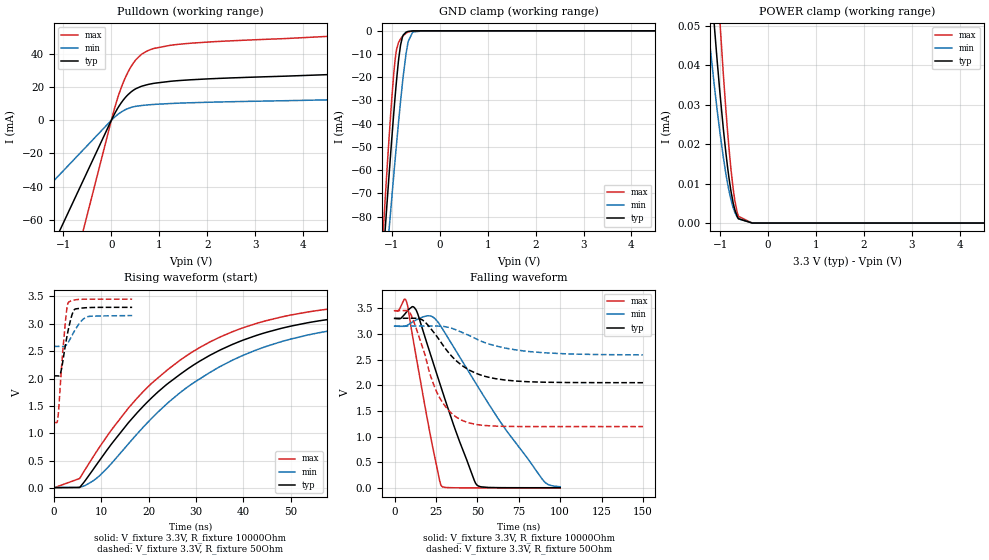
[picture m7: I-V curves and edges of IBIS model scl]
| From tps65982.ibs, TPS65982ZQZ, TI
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|   scl Model
[Model]   scl
Model_type   I/O_open_drain
Polarity   Non-Inverting
Vinl = 0.80
Vinh = 2.00
Vmeas = 1.65
Vref = 3.3
Cref = 2pF
Rref = 10000
|   typ   min   max
|   (nom PVT)   (fast PVT)   (slow PVT)
C_comp   8.631e-13   8.505e-13   8.892e-13
| Where nom  PVT is Nominal Process, 3.3V, 27C
|   Fast PVT is Strong Process,  3.45V, -40C
|   Slow PVT is Weak Process,   3.15V, 125C
[Voltage Range]   3.3   3.15   3.45
|Junction Temperature
[Temperature Range]   27   125   -40
[Pullup Reference]   3.3   3.15   3.45
[Pulldown Reference]   0   0   0
[Power Clamp Reference]   3.3   3.15   3.45
[GND Clamp Reference]   0   0   0
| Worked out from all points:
|   slope of the pulldown table from 0 to 0.495 V, typ, clamps not added: 26.4 ohm
|   GND clamp passes 1 mA (typ) near -0.72 V on its own axis
|   falling waveform, V_fixture 3.3V, R_fixture 10000Ohm: 20-80 % time 20.9ns typ, 38.8ns min, 11.8ns max; typ from 3.3 V to 0.005 V
|   rising waveform, V_fixture 3.3V, R_fixture 10000Ohm: 20-80 % time 26.8ns typ, 28.1ns min, 25.7ns max; typ from 0.005 V to 3.28 V
|   falling waveform, V_fixture 3.3V, R_fixture 50Ohm: 20-80 % time 21.7ns typ, 30.6ns min, 15.2ns max; typ from 3.3 V to 2.05 V
|   rising waveform, V_fixture 3.3V, R_fixture 50Ohm: 20-80 % time 1.6ns typ, 2.37ns min, 1.21ns max; typ from 2.05 V to 3.3 V
[Pulldown]
|   Voltage   I(typ)   I(min)   I(max)
-3.3V     -204.1mA   -100.3mA   -374.1mA
-55.5mV   -3.433mA   -1.687mA   -6.291mA
63.75mV   3.72mA     1.782mA    6.922mA
132.8mV   7.276mA    3.46mA     13.56mA
308.7mV   14.28mA    6.613mA    26.84mA
412.2mV   17.12mA    7.756mA    32.46mA
519.2mV   19.17mA    8.464mA    36.77mA
753.8mV   21.53mA    9.255mA    41.92mA
1.251V    23.57mA    10.13mA    45.33mA
1.645V    24.41mA    10.56mA    46.48mA
5.363V    28.43mA    12.81mA    51.9mA
6.6V      30.97mA    14.1mA     56.05mA
[GND Clamp]
|   Voltage   I(typ)   I(min)   I(max)
-3.3V     -769.8mA   -681.9mA   -862.9mA
-1.224V   -111.3mA   -127.9mA   -102mA
-1.109V   -77.43mA   -98.96mA   -63.21mA
-1.051V   -60.73mA   -84.56mA   -44.53mA
-964.4mV  -37.15mA   -63.69mA   -19.94mA
-912.3mV  -24.19mA   -51.54mA   -9.676mA
-815.1mV  -5.994mA   -30.18mA   -3.458mA
-701.3mV  -575.2uA   -9.847mA   -1.031mA
-653.9mV  -240.8uA   -4.467mA   -490.7uA
-562.6mV  -38.43uA   -514.1uA   -74.23uA
-330mV    -101.2nA   -940.3nA   -65.96nA
6.6V      0A         0A         0A
[POWER Clamp]
|   Voltage   I(typ)   I(min)   I(max)
-3.3V     548.7uA    403.1uA    721.8uA
-1.299V   79.98uA    55.9uA     116.4uA
-1.208V   64.23uA    44.79uA    94.82uA
-1.111V   48.63uA    33.84uA    73.12uA
-1.004V   33.07uA    23.01uA    51.08uA
-881.5mV  18.07uA    12.69uA    29.13uA
-815.1mV  11.51uA    8.232uA    19.09uA
-774.6mV  8.211uA    6.002uA    13.83uA
-695.3mV  3.499uA    2.796uA    5.93uA
-615.9mV  1.099uA    1.051uA    1.702uA
-330mV    0A         10.54nA    0A
6.6V      0A         0A         0A
[Ramp]
R_load = 10000
|   typ   min   max
dV/dt_r   1.96448/2.6802e-08   1.86581/2.80237e-08   2.05933/2.56593e-08
dV/dt_f   1.97678/2.08974e-08   1.87506/3.88653e-08   2.06819/1.17648e-08
[Falling Waveform]
V_fixture = 3.3V
V_fixture_min = 3.15V
V_fixture_max = 3.45V
R_fixture = 10000Ohm
|   Time   V(typ)   V(min)   V(max)
0s        3.3V       3.15V      3.45V
2.424ns   3.294V     3.145V     3.453V
5.864ns   3.371V     3.145V     3.673V
7.472ns   3.433V     3.162V     3.6V
13.1ns    3.458V     3.27V      2.544V
22.06ns   2.561V     3.344V     951.2mV
28.37ns   1.93V      3.124V     36.96mV
49.63ns   59.91mV    2.007V     3.042mV
89.15ns   5.387mV    171.7mV    3.011mV
100ns     5.367mV    24.9mV     3.011mV
[Rising Waveform]
V_fixture = 3.3V
V_fixture_min = 3.15V
V_fixture_max = 3.45V
R_fixture = 10000Ohm
|   Time   V(typ)   V(min)   V(max)
0s        5.363mV    10.67mV    3.011mV
5.446ns   9.254mV    13.61mV    173.8mV
8.292ns   337.1mV    130.9mV    567.9mV
15.68ns   1.186V     800.7mV    1.453V
20.71ns   1.652V     1.277V     1.917V
28.4ns    2.184V     1.856V     2.438V
37.73ns   2.624V     2.336V     2.855V
47.92ns   2.914V     2.671V     3.122V
60.42ns   3.108V     2.903V     3.293V
100ns     3.28V      3.12V      3.435V
[Falling Waveform]
V_fixture = 3.3V
V_fixture_min = 3.15V
V_fixture_max = 3.45V
R_fixture = 50Ohm
|   Time   V(typ)   V(min)   V(max)
0s        3.3V       3.15V      3.45V
9.336ns   3.303V     3.152V     3.409V
16.83ns   3.27V      3.152V     2.741V
21.34ns   3.123V     3.152V     2.222V
25.89ns   2.933V     3.15V      1.838V
32.75ns   2.629V     3.124V     1.508V
40.62ns   2.386V     3.029V     1.319V
55.51ns   2.165V     2.817V     1.214V
78.52ns   2.071V     2.665V     1.196V
150ns     2.049V     2.59V      1.195V
[Rising Waveform]
V_fixture = 3.3V
V_fixture_min = 3.15V
V_fixture_max = 3.45V
R_fixture = 50Ohm
|   Time   V(typ)   V(min)   V(max)
0s        2.049V     2.587V     1.195V
870ps     2.047V     2.587V     1.287V
1.418ns   2.098V     2.587V     1.944V
2.268ns   2.515V     2.59V      2.87V
2.73ns    2.749V     2.622V     3.261V
3.064ns   2.895V     2.664V     3.388V
3.8ns     3.154V     2.78V      3.423V
4.524ns   3.269V     2.894V     3.438V
7.212ns   3.296V     3.132V     3.45V
16.54ns   3.3V       3.15V      3.45V
